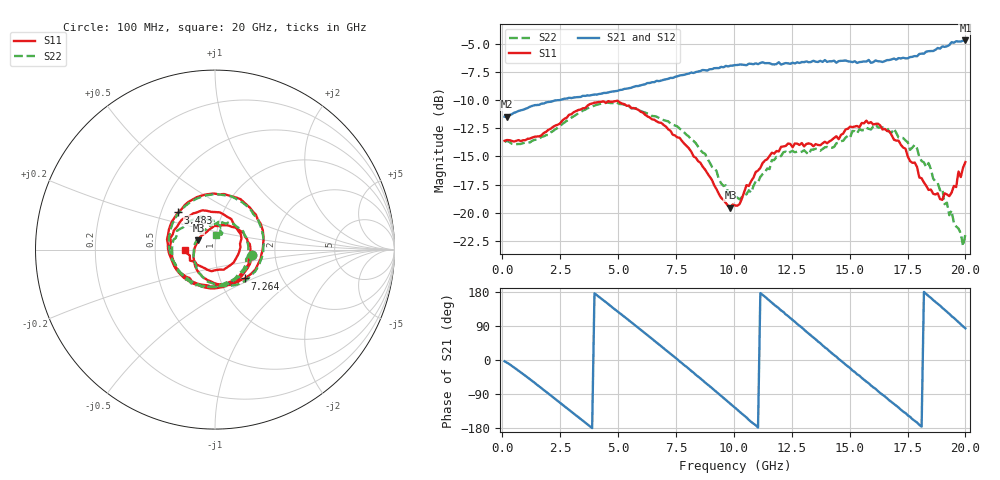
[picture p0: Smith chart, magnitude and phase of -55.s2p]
!Agilent Technologies,N5230C,MY49001569,A.09.33.09
!Agilent N5230C: A.09.33.09
!Date: Monday, July 27, 2015 20:14:56
!Correction: S11(Full 2 Port(1,2))
!S21(Full 2 Port(1,2))
!S12(Full 2 Port(1,2))
!S22(Full 2 Port(1,2))
!S2P File: Measurements: S11, S21, S12, S22:
# Hz S  dB  R 50
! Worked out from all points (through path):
!   201 points, 100 MHz to 20 GHz, reference 50 ohm
!   highest |S21| = -4.67 dB at 20 GHz (marker M1); lowest = -11.5 dB at 199.5 MHz (marker M2)
!   group delay of S21, straight-line fit = 140 ps
!   lowest |S11| = -19.6 dB at 9.851 GHz (marker M3), VSWR 1.24, Z = 41.4 + j4.28 ohm
!   |S11| at or under -10 dB: start of sweep to end of sweep
!   |S22| runs from -23.0 to -10.2 dB; largest |S21 - S12| = 0.02
!   S11 on the Smith chart (normalised r, x): 100 MHz: 1.52, -0.09; 3.483 GHz: 0.61, +0.28; 7.264 GHz: 1.31, -0.45; 20 GHz: 0.71, -0.00
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1e8  -13.60 -8.0  -11.46 -3.3  -11.59 -3.0  -13.69 -8.0
1.995e8  -13.54 -15.0  -11.46 -6.8  -11.42 -6.8  -13.62 -15.4
1.5925e9  -13.21 -110.8  -10.40 -69.6  -10.34 -69.6  -13.43 -108.9
2.5875e9  -11.81 -175.1  -9.91 -117.4  -9.90 -117.7  -12.11 -171.3
3.483e9  -10.71 134.7  -9.60 -160.4  -9.62 -160.4  -10.91 138.7
4.3785e9  -10.10 90.7  -9.35 157.0  -9.37 156.5  -10.28 95.5
5.3735e9  -10.49 44.9  -8.96 109.2  -8.96 108.6  -10.43 51.5
6.7665e9  -11.98 -21.1  -8.29 41.1  -8.26 40.7  -11.57 -10.6
7.264e9  -12.72 -44.0  -8.00 16.1  -8.02 16.0  -12.07 -33.0
8.458e9  -15.42 -109.8  -7.44 -43.9  -7.42 -44.2  -14.13 -87.5
9.851e9  -19.55 150.9  -6.92 -115.6  -6.99 -116.2  -18.44 -172.9
1.005e10  -19.36 133.1  -6.86 -125.9  -6.88 -126.9  -18.58 171.1
1.1443e10  -15.24 38.8  -6.69 161.7  -6.73 160.9  -16.07 75.2
1.25375e10  -14.18 -16.0  -6.65 105.8  -6.64 105.3  -14.51 18.3
1.3433e10  -14.09 -67.0  -6.48 59.5  -6.66 59.3  -14.39 -28.4
1.4826e10  -12.59 -147.7  -6.45 -12.2  -6.57 -13.0  -13.32 -104.6
1.5821e10  -12.04 160.2  -6.40 -61.3  -6.58 -63.1  -12.54 -154.3
1.67165e10  -12.76 108.2  -6.41 -106.7  -6.34 -107.0  -12.82 163.9
1.75125e10  -15.00 54.5  -6.26 -146.1  -6.12 -146.6  -13.74 125.7
1.8408e10  -17.98 -26.8  -5.63 168.7  -5.67 168.6  -15.58 86.7
1.9204e10  -18.39 -113.6  -5.19 127.2  -5.03 127.0  -19.11 75.0
2e10  -15.50 -179.5  -4.67 83.7  -4.62 82.7  -21.93 85.9
